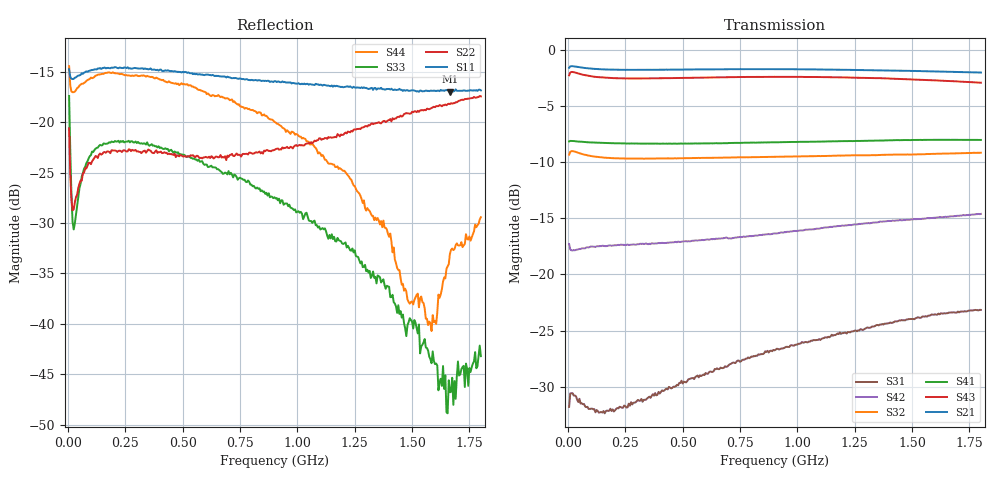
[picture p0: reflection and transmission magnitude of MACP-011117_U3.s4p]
!Agilent Technologies,E5071C,MY46630996,B.13.30
!Date: Tue Jan 23 09:28:35 2024
!Data & Calibration Information:
!MACP-011117 soldered onto PT-0013779 with F connectors, Calibration PT-0003645-TRL. Port1 (pin1) Port2 (pin5) Port3 (pin4) Port4 (pin3)
!Freq	S11:SOLT4(ON)	S12:SOLT4(ON)	S13:SOLT4(ON)	S14:SOLT4(ON)
!	S21:SOLT4(ON)	S22:SOLT4(ON)	S23:SOLT4(ON)	S24:SOLT4(ON)
!	S31:SOLT4(ON)	S32:SOLT4(ON)	S33:SOLT4(ON)	S34:SOLT4(ON)
!	S41:SOLT4(ON)	S42:SOLT4(ON)	S43:SOLT4(ON)	S44:SOLT4(ON)
!PortZ  Port1:75+j0  Port2:75+j0  Port3:75+j0  Port4:75+j0
!Above PortZ is port z conversion or system Z0 setting when saving the data.
!When reading, reference impedance value at option line is always used.
# Hz S MA R 75
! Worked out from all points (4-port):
!   360 points, 5 MHz to 1.8 GHz, reference 75 ohm
!   strongest paths, dB at 5 MHz, 455 MHz, 905 MHz, 1.355 GHz, 1.8 GHz:
!     S21: -1.6, -1.8, -1.7, -1.8, -2.0
!     S43: -2.3, -2.5, -2.4, -2.5, -2.9
!     S41: -8.2, -8.4, -8.2, -8.1, -8.0
!     S32: -9.3, -9.7, -9.5, -9.4, -9.2
!     S42: -17.3, -17.1, -16.4, -15.3, -14.6
!     S31: -31.8, -30.1, -26.7, -24.5, -23.2
!   lowest |S11| = -17.0 dB at 1.665 GHz (marker M1), VSWR 1.33, Z = 56.7 + j3.63 ohm
!   |S11| at or under -10 dB: start of sweep to end of sweep
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5000000  0.1836 163.7  0.8325 3.6  0.02727 27.2  0.3891 -178.3
         0.8309 3.7  0.09343 128.2  0.3393 8.7  0.1361 173.1
         0.02574 21.3  0.3411 8.6  0.1353 119.3  0.7706 6.8
         0.3909 -178.1  0.1366 173.6  0.7699 6.6  0.1901 153.0
2.5e7  0.1645 178.9  0.8441 -0.3  0.02893 1.7  0.3923 178.6
       0.8439 -0.3  0.03695 175.4  0.3532 0.3  0.1279 178.0
       0.02893 2.1  0.353 0.3  0.0294 165.8  0.7941 -0.4
       0.3923 178.6  0.1284 178.1  0.7944 -0.4  0.1413 177.2
1.55e8  0.1864 179.9  0.8177 -3.3  0.02465 5.7  0.3848 170.6
        0.8175 -3.4  0.07105 -165.6  0.3313 -2.8  0.1339 173.9
        0.02466 6.3  0.331 -2.8  0.07858 -170.2  0.7518 -5.6
        0.3846 170.6  0.134 173.7  0.7517 -5.6  0.1742 173.3
7e8  0.1676 168.8  0.8195 -11.7  0.03781 22.3  0.3835 141.2
     0.8193 -11.7  0.06738 -153.6  0.3316 -5.4  0.1462 148.0
     0.03941 22.7  0.3312 -5.3  0.05731 157.3  0.7552 -19.6
     0.3846 141.3  0.1446 147.0  0.7555 -19.6  0.131 131.6
1.585e9  0.1436 166.7  0.7992 -27.8  0.06041 0.3  0.3937 93.9
         0.8015 -28.0  0.118 -127.0  0.3442 -13.7  0.1808 103.7
         0.06632 1.6  0.3437 -13.5  0.006373 174.9  0.7322 -49.3
         0.397 94.0  0.1784 102.1  0.7322 -49.3  0.009208 -20.6
1.665e9  0.1419 167.2  0.7959 -29.2  0.06171 -3.5  0.3943 89.8
         0.7978 -29.4  0.1232 -126.7  0.3451 -14.6  0.183 99.7
         0.06762 -2.4  0.3452 -14.5  0.004573 -139.1  0.7255 -52.1
         0.3974 89.8  0.1813 98.3  0.7253 -52.1  0.02222 -67.2
1.8e9  0.1442 168.2  0.7913 -31.7  0.0642 -9.1  0.3942 82.6
       0.7919 -31.9  0.1346 -126.2  0.3477 -16.3  0.1884 93.2
       0.06951 -8.2  0.3481 -16.1  0.006908 -76.0  0.7124 -57.1
       0.3969 82.7  0.1859 91.8  0.7133 -57.1  0.03383 -87.9
